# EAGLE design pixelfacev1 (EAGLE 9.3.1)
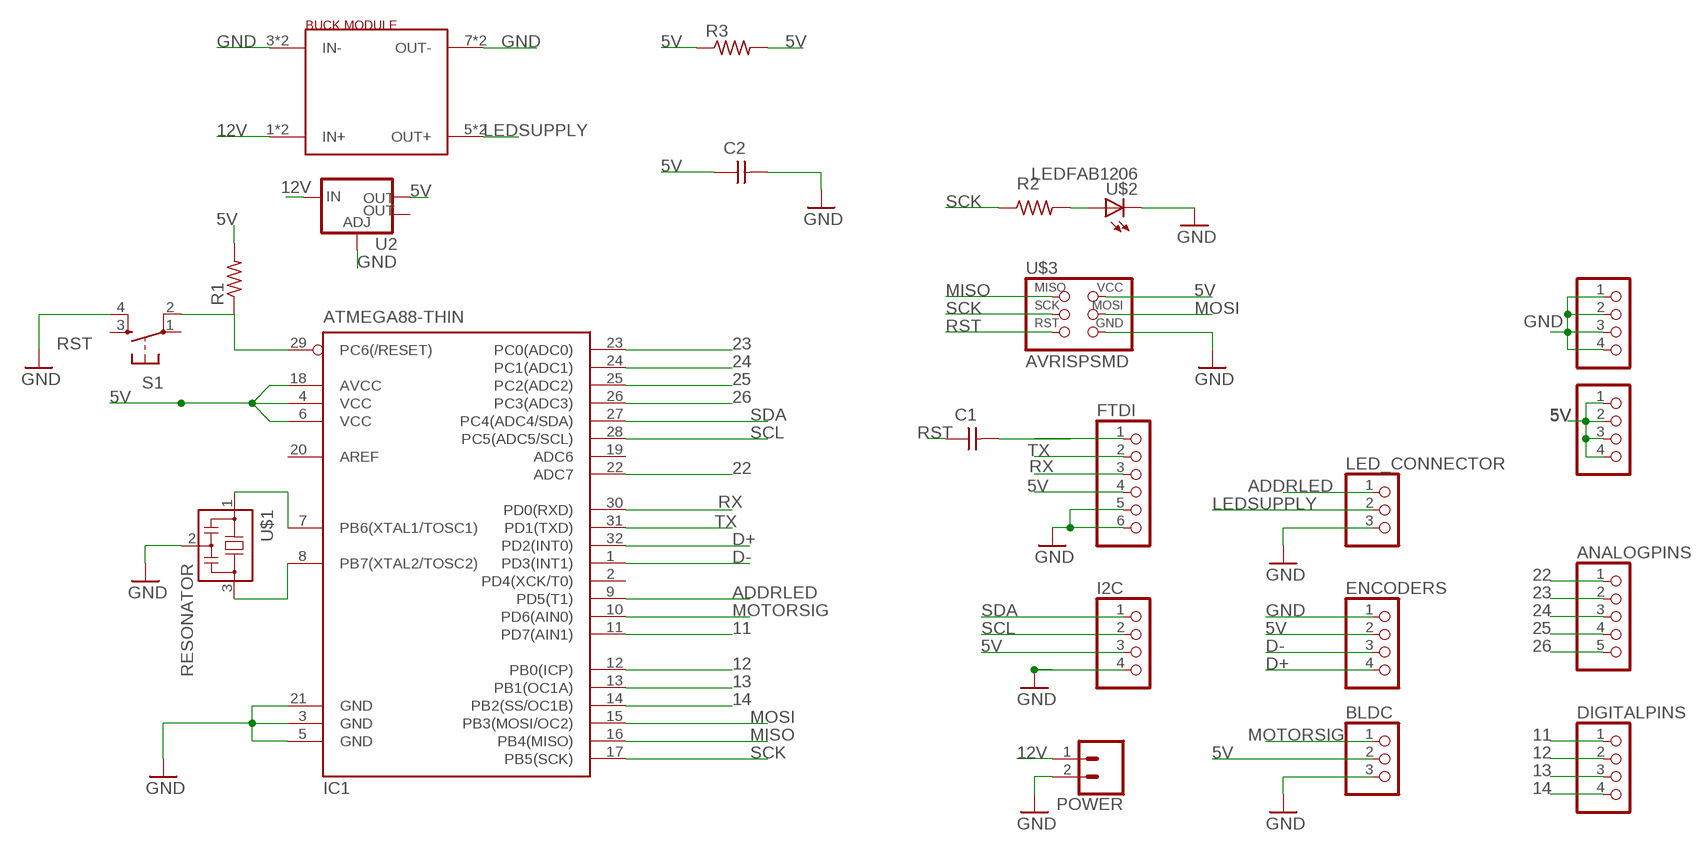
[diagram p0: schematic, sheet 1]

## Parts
5V  PINHD-1X41X04_SMT  [1X04_SMT]
ANALOGPINS  PINHD-1X51X05_SMT  [1X05_SMT]
BLDC  PINHD-1X31X03_SMT  [1X03_SMT]
C1  CAP-UNPOLARIZEDFAB  [C1206FAB]
C2  CAP-UNPOLARIZEDFAB  [C1206FAB]
DIGITALPINS  PINHD-1X41X04_SMT  [1X04_SMT]
ENCODERS  PINHD-1X41X04_SMT  [1X04_SMT]
FTDI  PINHD-1X61X06_SMT  [1X06_SMT]
GND  PINHD-1X41X04_SMT  [1X04_SMT]
I2C  PINHD-1X41X04_SMT  [1X04_SMT]
IC1  ATMEGA88-THIN  [TQFP32-08THIN]
LED_CONNECTOR  PINHD-1X31X03_SMT  [1X03_SMT]
POWER  CONN_02PTH4  [1X02_XTRA_BIG]
R1  RES-US1206FAB  [R1206FAB]
R2  RES-US1206FAB  [R1206FAB]
R3  RES-US1206FAB  [R1206FAB]
S1  6MM_SWITCH6MM_SWITCH  [6MM_SWITCH]
U2  V_REG_LM1117SOT223  [SOT223]
U$1  RESONATOR  [EFOBM]
U$2  LEDFAB1206  [LED1206FAB]
U$3  AVRISPSMD  [2X03SMD]
U$4  GENERIC_BUCK_MODULE  [GENERIC_BUCK_MODULE]

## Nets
5V: 5V.1 5V.2 5V.3 5V.4 BLDC.2 C2.1 ENCODERS.2 FTDI.4 I2C.3 IC1.4(VCC) IC1.6(VCC) IC1.18(AVCC) R1.2 R3.1 R3.2 U2.2(OUT) U$3.2(VCC)
11: DIGITALPINS.1 IC1.11(PD7(AIN1))
12: DIGITALPINS.2 IC1.12(PB0(ICP))
12V: POWER.1 U2.3(IN) U$4.1(IN+) U$4.2(IN+)
13: DIGITALPINS.3 IC1.13(PB1(OC1A))
14: DIGITALPINS.4 IC1.14(PB2(SS/OC1B))
22: ANALOGPINS.1 IC1.22(ADC7)
23: ANALOGPINS.2 IC1.23(PC0(ADC0))
24: ANALOGPINS.3 IC1.24(PC1(ADC1))
25: ANALOGPINS.4 IC1.25(PC2(ADC2))
26: ANALOGPINS.5 IC1.26(PC3(ADC3))
ADDRLED: IC1.9(PD5(T1)) LED_CONNECTOR.1
D+: ENCODERS.4 IC1.32(PD2(INT0))
D-: ENCODERS.3 IC1.1(PD3(INT1))
GND: BLDC.3 C2.2 ENCODERS.1 FTDI.5 FTDI.6 GND.1 GND.2 GND.3 GND.4 I2C.4 IC1.3(GND) IC1.5(GND) IC1.21(GND) LED_CONNECTOR.3 POWER.2 S1.4(S1) U2.1(ADJ) U$1.2 U$2.2(C) U$3.6(GND) U$4.3(IN-) U$4.4(IN-) U$4.7(OUT-) U$4.8(OUT-)
LEDSUPPLY: LED_CONNECTOR.2 U$4.5(OUT+) U$4.6(OUT+)
MISO: IC1.16(PB4(MISO)) U$3.1(MISO)
MOSI: IC1.15(PB3(MOSI/OC2)) U$3.4(MOSI)
MOTORSIG: BLDC.1 IC1.10(PD6(AIN0))
N$1: IC1.7(PB6(XTAL1/TOSC1)) U$1.1
N$2: IC1.8(PB7(XTAL2/TOSC2)) U$1.3
N$4: R2.2 U$2.1(A)
N$6: C1.2 FTDI.1
RST: C1.1 IC1.29(PC6(/RESET)) R1.1 S1.2(P1) U$3.5(RST)
RX: FTDI.3 IC1.30(PD0(RXD))
SCK: IC1.17(PB5(SCK)) R2.1 U$3.3(SCK)
SCL: I2C.2 IC1.28(PC5(ADC5/SCL))
SDA: I2C.1 IC1.27(PC4(ADC4/SDA))
TX: FTDI.2 IC1.31(PD1(TXD))
Unconnected: IC1.2(PD4(XCK/T0)) IC1.19(ADC6) IC1.20(AREF) S1.1(P) S1.3(S) U2.4(OUT)

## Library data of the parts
5V DIGITALPINS ENCODERS GND I2C = smd_con:PINHD-1X4: PIN HEADER
ANALOGPINS = smd_con:PINHD-1X5: PIN HEADER
BLDC LED_CONNECTOR = smd_con:PINHD-1X3: PIN HEADER
C1 C2 = fab:CAP-UNPOLARIZED
FTDI = smd_con:PINHD-1X6: PIN HEADER
IC1 = fab:ATMEGA88-THIN
POWER = SparkFun-Connectors:CONN_02: Multi connection point. Often used as Generic Header-pin footprint for 0.1 inch spaced/style header connections
R1-R3 = fab:RES-US: Resistor (US Symbol)
S1 = fab:6MM_SWITCH: OMRON SWITCH
U2 = fab:V_REG_LM1117: Voltage Regulator LM1117 Standard adjustable voltage regulator but in SMD form. Spark Fun Electronics SKU : COM-00595; PROD_ID: VREG-08170
U$1 = fab:RESONATOR
U$2 = fab:LED: LED
U$3 = fab:AVRISP
U$4 = CN1584:GENERIC_BUCK_MODULE

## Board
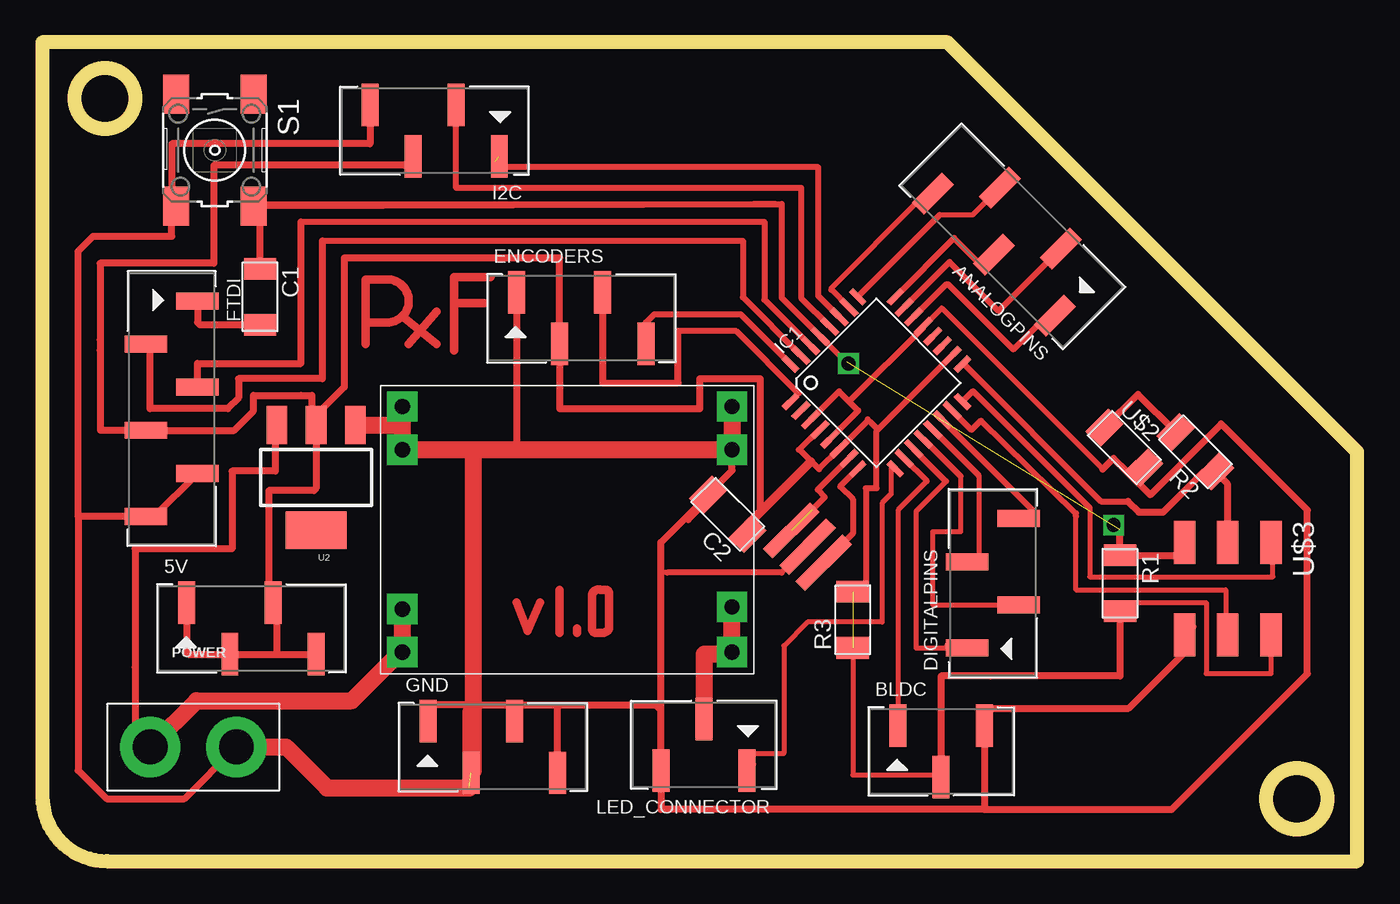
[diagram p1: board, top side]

Size 77.47 x 48.26 mm. Coordinates in mm from the lower left corner, seen from the top.
Outline: 3.81,0 77.47,0 77.47,24.13 53.34,48.26 0,48.26 0,3.81 arc90 3.81,0
Outline: circle at 3.68,44.96 radius 1.8
Outline: circle at 73.91,3.68 radius 1.8
Copper layers (1*16): Top 0.035mm / dielectric 1.5mm / Bottom 0.035mm
Design rules "default *": minimum track width 6mil, minimum drill 0.35mm, track to track 15mil, track to pad 12mil, pad to pad 8mil, via to via 16mil, smd to smd 15mil, copper to edge 40mil, drill to drill 32mil, minimum pad ring 10mil, minimum via ring 8mil, stop-mask expansion 4mil, vias tented up to drill 0mil, thermal gap 10mil

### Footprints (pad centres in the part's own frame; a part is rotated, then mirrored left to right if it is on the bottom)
1X04_SMT = smd 1 x 2.5: 1 -3.81,1.52; 2 -1.27,-1.52; 3 1.27,1.52; 4 3.81,-1.52
1X05_SMT = smd 1 x 2.5: 1 -5.08,1.52; 2 -2.54,-1.52; 3 0,1.52; 4 2.54,-1.52; 5 5.08,1.52
1X03_SMT = smd 1 x 2.5: 1 -2.54,1.52; 2 0,-1.52; 3 2.54,1.52
C1206FAB = smd 1.27 x 1.905: 1 -1.651,0; 2 1.651,0
1X06_SMT = smd 1 x 2.5: 1 -6.35,1.52; 2 -3.81,-1.52; 3 -1.27,1.52; 4 1.27,-1.52; 5 3.81,1.52; 6 6.35,-1.52
TQFP32-08THIN = smd 1.118 x 0.356: 1 -4.369,2.8; 8 -4.369,-2.8; 17 4.369,-2.8; 24 4.369,2.8 | smd 1.27 x 0.356: 2 -4.293,2; 3 -4.293,1.2; 4 -4.293,0.4; 5 -4.293,-0.4; 6 -4.293,-1.2; 7 -4.293,-2; 18 4.293,-2; 19 4.293,-1.2; 20 4.293,-0.4; 21 4.293,0.4; 22 4.293,1.2; 23 4.293,2 | smd 0.356 x 1.118: 9 -2.8,-4.369; 16 2.8,-4.369; 25 2.8,4.369; 32 -2.8,4.369 | smd 0.356 x 1.27: 10 -2,-4.293; 14 1.2,-4.293; 15 2,-4.293; 26 2,4.293; 27 1.2,4.293; 31 -2,4.293 | smd 0.35 x 1.27: 11 -1.2,-4.293; 12 -0.4,-4.293; 13 0.4,-4.293; 28 0.4,4.293; 29 -0.4,4.293; 30 -1.2,4.293
1X02_XTRA_BIG = drill 2.057 pad 3.556: 1 -2.54,0; 2 2.54,0
R1206FAB = smd 1.27 x 1.905: 1 -1.651,0; 2 1.651,0
6MM_SWITCH = smd 2.286 x 1.524: 1 -3.302,2.286; 2 3.302,2.286; 3 -3.302,-2.286; 4 3.302,-2.286
SOT223 = smd 1.219 x 2.235: 1 -2.311,-3.099; 2 0,-3.099; 3 2.311,-3.099 | smd 3.6 x 2.2: 4 0,3.099
EFOBM = smd 0.8 x 3.9: 1 -1.35,0; 2 0,0; 3 1.35,0
LED1206FAB = smd 1.27 x 1.905: 1 -1.651,0; 2 1.651,0
2X03SMD = smd 2.54 x 1.27: 1 -2.54,2.54; 2 2.92,2.54; 3 -2.54,0; 4 2.92,0; 5 -2.54,-2.54; 6 2.92,-2.54
GENERIC_BUCK_MODULE = drill 0.9 pad 1.778 square: 1 1.27,1.27; 2 1.27,3.81; 3 1.27,13.208; 4 1.27,15.748; 5 20.701,1.27; 6 20.701,3.937; 7 20.701,13.208; 8 20.701,15.748

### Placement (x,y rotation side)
5V  12.32,13.72 0 top
ANALOGPINS  57.15,36.83 135 top
BLDC  52.96,6.48 0 top
C1  12.83,33.27 270 top
C2  40.39,20.45 135 top
DIGITALPINS  56.01,16.38 90 top
ENCODERS  31.75,32 0 top
FTDI  7.62,26.67 270 top
GND  26.54,6.73 0 top
I2C  23.11,43.05 180 top
IC1  49.15,28.19 45 top
LED_CONNECTOR  38.99,6.86 180 top
POWER  8.89,6.73 0 top
R1  63.5,16.38 270 top
R2  67.94,24.13 135 top
R3  47.75,14.22 90 top
S1  10.16,41.91 270 top
U2  16.13,22.61 180 top
U$1  45.08,18.54 315 top
U$2  63.75,24.38 315 top
U$3  69.85,16.26 270 top
U$4  19.94,11.05 0 top

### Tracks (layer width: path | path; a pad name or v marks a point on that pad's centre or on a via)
5V  (1 unrouted)
  Top 0.305: U$3.2 72.39,11.05 68.58,11.05 68.58,15.24 64.01,15.24 R1.2 | 49.15,25.37 49.23,25.45 IC1.18 | 48.64,26.04 48.77,25.91 | 48.51,15.88 R3.2 | R3.1 47.75,5.08 52.96,5.08 | 45.77,23.11 45.72,23.11 45.28,23.56 44.58,24.26 45.76,25.44 IC1.4
  Top 0.356: 48.64,26.04 48.64,25.99 IC1.6 45.77,23.11 44.62,24.26 | 44.62,24.26 44.58,24.26 | 44.62,24.26 45.81,25.44 IC1.4 | 48.77,25.91 49.23,25.45 | IC1.18 49.15,25.37 49.15,21.97 48.51,21.97 48.51,15.88
  Top 0.406: 3.4,30.73 3.4,35.25 10.1,35.25 10.1,41.02 21.33,41.02 I2C.3 | 3.4,30.73 3.4,30.11 | 16.13,26.29 U2.2 16.13,21.97 16,21.84 13.33,21.84 13.33,15.49 5V.3 13.84,14.98 13.84,12.32 13.97,12.2 | 16.13,26.29 17.78,27.94 17.78,35.56 30.48,35.56 ENCODERS.2 30.48,26.67 38.73,26.67 38.73,28.45 42.29,28.45 42.29,20.57 42.16,20.45 | 63.86,15.09 R1.2 63.5,10.92 55.88,10.92 52.96,10.92 52.96,5.08 BLDC.2 | C2.1 41.55,19.79 | 3.4,30.73 3.43,30.71 3.43,25.4 FTDI.4 11.3,25.4 12.45,26.54 12.45,27.46 15.24,27.46 15.88,27.46 15.88,26.54 16.13,26.29 | 5V.1 8.51,12.32 8.63,12.2 5V.2 13.97,12.2 | 13.97,12.2 5V.4
  Top 0.508: C2.1 41.55,19.84 42.16,20.45 45.28,23.56
11
  Top 0.305: 53.25,22.39 51.49,20.62 51.49,12.57 DIGITALPINS.1
  Top 0.356: IC1.11 53.25,22.39
  Top 0.406: DIGITALPINS.1 54.36,12.7 53.34,12.7
12
  Top 0.305: 54.1,22.7 54.1,19.43 52.45,19.43 52.45,15.11 DIGITALPINS.2
  Top 0.356: IC1.12 54.1,22.7
12V
  Top 0.406: U2.3 13.82,25.25 13.72,25.15 13.72,22.99 11.18,22.99 11.18,18.41 5.46,18.41 5.46,11.43 5.46,7.87 6.48,6.86
  Top 0.813: U$4.1 21.08,12.32
  Top 1.016: 21.08,12.32 18.22,9.46 9.08,9.46 6.48,6.86 POWER.1 | U$4.2 U$4.1
13
  Top 0.305: 55.18,22.73 55.18,17.58
  Top 0.356: IC1.13 55.18,22.73
  Top 0.406: 55.18,17.58 55.1,17.65 DIGITALPINS.3
14
  Top 0.305: 58.42,20.62 58.42,20.32 58.42,20.19
  Top 0.356: IC1.14 58.42,20.62
  Top 0.406: DIGITALPINS.4 58.29,20.19 58.42,20.32
22
  Top 0.305: 59.18,31.88 59.47,32.16 ANALOGPINS.1
  Top 0.356: IC1.22 53.27,34.01 53.36,34.01 57.21,30.16 58.93,31.88 59.18,31.88
23
  Top 0.254: 59.45,35.54 59.58,35.67
  Top 0.305: ANALOGPINS.2 59.58,35.67 | ANALOGPINS.2
  Top 0.356: IC1.23 53.45,35.32 56.34,32.43 59.45,35.54 | 59.45,35.54
  Top 0.406: ANALOGPINS.2 60.02,36.02
24
  Top 0.305: 55.27,35.18 55.5,35.18 ANALOGPINS.3
  Top 0.356: IC1.24 53.72,36.73 55.27,35.18
25
  Top 0.305: ANALOGPINS.4 54.83,38.1 52.88,38.1
  Top 0.356: IC1.25 52.88,38.1
26
  Top 0.305: 46.48,33.69 46.48,33.78 51.69,38.99 52.12,38.99 ANALOGPINS.5
  Top 0.356: IC1.26 46.48,33.69
ADDRLED
  Top 0.305: IC1.9 50,23.12 50,21.64 49.48,21.11 49.48,14.1 45.08,14.1 43.69,12.7 43.69,6.35 41.91,6.35 41.91,5.72 LED_CONNECTOR.1
D+
  Top 0.305: ENCODERS.4 35.56,31.75
  Top 0.356: IC1.32 41.14,32.25 36.06,32.25 35.56,31.75
D-
  Top 0.305: IC1.1 44.57,27.57
  Top 0.356: 37.47,31.24 40.89,31.24 44.57,27.57
  Top 0.406: ENCODERS.3 33.02,28.19 37.47,28.19 37.47,31.24
GND  (1 unrouted)
  Top 0.254: 46.94,27.69 47.54,27.09 | 48.06,26.57 47.54,27.09 | IC1.21 47.54,27.15 47.54,27.09
  Top 0.305: 62.48,23.11 52.99,32.6 IC1.21 51.9,31.45 | U$1.2 43.56,17.02 | 36.83,17.02 36.45,17.02 | S1.4 7.87,38.1 | C2.2 39.2,21.6 39.2,21.3
  Top 0.356: IC1.3 46.94,27.69 48.06,26.57 48.06,26.54 IC1.5 | 47.54,27.15 47.6,27.15 51.9,31.45 | 43.56,17.02 36.83,17.02
  Top 0.406: 2.11,20.32 2.11,5.35 3.77,3.68 8.38,3.68 POWER.2 | U$3.6 67.63,13.65 | 67.63,13.65 67.79,13.82 | 64.92,23.52 U$2.2 | 39.2,21.3 38.05,20.14 | 27.94,24.13 25.4,24.13 21.21,24.13 U$4.3 21.21,25.65 | 40.64,24.13 27.94,24.13 | 40.64,24.13 40.64,23.04 C2.2 39.22,21.57 36.45,18.8 36.45,17.02 36.45,8.89 | 40.64,24.13 U$4.7 | U2.1 18.44,25.4 | FTDI.5 6.6,20.32 FTDI.6 2.11,20.32 | 19.18,44.45 I2C.4 19.3,42.29 7.62,42.29 7.62,38.35 | 2.11,20.32 2.11,35.96 2.98,36.83 7.62,36.83 7.62,38.35 | 55.5,3.05 36.45,3.05 LED_CONNECTOR.3 36.45,8.89 | 55.5,3.05 BLDC.3 55.5,8.89 55.37,9.02 64.01,9.02 67.31,12.32 67.31,12.7 67.63,13.02 67.63,13.65 | 25.4,9.22 27.94,9.22 | 27.94,9.22 30.48,9.22 | 30.48,9.22 36.12,9.22 36.45,8.89 | 25.27,8.89 25.27,9.09 25.4,9.22 | GND.4 30.35,9.09 30.48,9.22 | 25.13,5.35 GND.2 | 25.4,9.22 22.81,9.22 22.73,9.14 GND.1 | GND.3 27.81,9.09 27.94,9.22 | ENCODERS.1 27.94,24.13 | 55.5,3.05 66.55,3.05 74.55,11.05 74.55,20.7 69.47,25.78 65.28,21.59 63.88,22.99 | U$2.2 64.95,23.24 | U$2.2 64.96,23.18 64.77,22.99 63.88,22.99 | 62.48,23.11 63.12,23.75 63.88,22.99 | 7.62,38.35 7.87,38.1 | 7.62,38.35 S1.4
  Top 1.016: U$4.4 21.21,25.65 | 21.21,25.65 21.21,24.13 | 18.57,25.27 18.44,25.4 | U$4.3 40.51,24.26 40.64,24.13 | U$4.8 U$4.7 | 25.4,9.02 25.27,8.89 GND.2 25.4,5.34 25.4,9.02 | 25.4,9.02 25.4,9.22 25.4,24.13 | U2.1 19.05,25.71 21.16,25.71 21.21,25.65 | POWER.2 14.35,6.73 16.76,4.32 25.15,4.32
LEDSUPPLY
  Top 0.813: U$4.5 40.51,12.19
  Top 1.016: LED_CONNECTOR.2 38.99,12.19 40.51,12.19 | U$4.5 U$4.6
MISO
  Top 0.305: 61.72,20.83 61.72,16.76 72.52,16.76 72.52,18.16 72.9,18.54 72.64,18.8 U$3.1
  Top 0.356: IC1.16 54.84,27.71 61.72,20.83
MOSI
  Top 0.305: 60.91,20.32 60.91,16 69.72,16 69.72,14.35 69.98,14.1 | U$3.4 70.1,13.59 70.1,13.97
  Top 0.356: IC1.15 54.75,25.42 55.31,25.97 60.91,20.5 60.91,20.32
  Top 0.406: 70.1,13.97 69.98,14.1
MOTORSIG
  Top 0.305: BLDC.1 50.42,20.7 52.12,22.4
  Top 0.356: IC1.10 52.12,22.4
N$1  (1 unrouted)
  Top 0.356: IC1.7 45.69,21.91 | 45.69,21.91 | 45.69,21.91 46.1,21.46 45.34,20.7
N$2
  Top 0.254: 47.75,19.3 47.12,18.67 | 47.12,18.66 47.12,18.28
  Top 0.305: 46.29,17.59 U$1.3
  Top 0.356: IC1.8 47,22.09 47.75,21.34 47.75,19.3 47.12,18.66
  Top 0.406: U$1.3 47.12,18.66 47.12,18.67
N$3  (via drill 0.81)
  other vias: 63.12,19.81
N$4
  Top 0.406: R2.2 64.55,27.52 U$2.1
N$5  (via drill 0.81)
  other vias: 47.5,29.34
N$6
  Top 0.406: FTDI.1 9.14,31.75 9.27,31.62 C1.2
N$7
  Top 0.508: 19.05,30.48 19.05,31.75 | 19.05,31.75 19.05,34.29 20.32,34.29 arc-90 21.59,33.02 arc-90 20.32,31.75 19.05,31.75
N$8
  Top 0.508: 21.59,30.48 23.24,32.39
N$9
  Top 0.508: 21.21,32.13 23.24,30.48
N$10
  Top 0.508: 24.26,30.1 24.26,34.42
N$11
  Top 0.508: 24.38,34.42 26.42,34.42
N$12
  Top 0.508: 24.38,32.89 26.04,32.89
N$13
  Top 0.508: 27.94,15.24 28.57,13.59 29.34,15.24
N$14
  Top 0.508: 30.48,16 30.48,13.46
N$15
  Top 0.508: 31.5,13.46 31.5,13.72
N$16
  Top 0.508: 32.38,13.72 32.38,15.62 arc-106 32.89,16 33.15,16 arc-90 33.4,15.75 33.4,13.84 arc-90 33.02,13.46 32.64,13.46 arc-90 32.38,13.72
RST  (1 unrouted)
  Top 0.305: 41.91,38.73 12.83,38.73 | IC1.29 47.31,29.46 47.37,29.46
  Top 0.356: IC1.29 43.56,33.22 43.56,38.73 | S1.2 43.18,38.73 | 43.18,38.73 41.91,38.73 | 43.18,38.73 43.56,38.73 | 43.56,38.73
  Top 0.406: C1.1 12.83,38.73 12.7,38.61 S1.2 | 63.5,19.56 R1.1 67.31,18.03 | 67.44,17.91 67.31,17.91 67.31,18.03 | U$3.5 67.31,18.03
RX
  Top 0.356: IC1.30 42.55,33.1 42.55,37.69 15.24,37.69
  Top 0.406: 15.24,37.69 15.24,29.34 9.14,29.34 FTDI.3
SCK
  Top 0.356: IC1.17 54.29,29.3 62.38,21.21 63.97,21.21
  Top 0.406: U$3.3 69.85,22.23 R2.1 68.43,22.96 66.04,20.57 64.61,20.57 63.97,21.21
SCL
  Top 0.305: 24.38,44.2 I2C.2
  Top 0.356: IC1.28 44.7,33.2 44.7,39.67 24.38,39.67 24.38,44.2
SDA  (1 unrouted)
  Top 0.356: IC1.27 45.72,33.32 45.72,40.89 26.67,40.89 26.67,41.27
  Top 0.406: 26.67,40.64 26.67,41.27 26.67,41.28
TX
  Top 0.356: IC1.31 41.27,33.24 41.27,36.58 16.51,36.58
  Top 0.406: 16.51,36.58 16.51,28.45 11.56,28.45 11.56,27.3 10.92,26.67 6.35,26.67 6.35,30.23 FTDI.2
